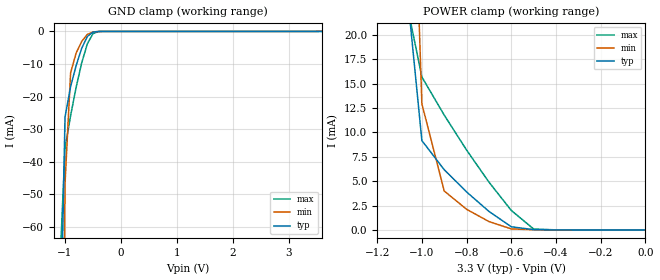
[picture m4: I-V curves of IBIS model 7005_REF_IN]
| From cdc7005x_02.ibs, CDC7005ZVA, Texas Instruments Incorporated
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| Device Control Input Receiver Model REF_IN
[Model]   7005_REF_IN
Model_type  Input
Polarity   Non-Inverting
Vinl = 0.8V
Vinh = 2.0V
| variable   typ   min   max
C_comp   0.57p   NA   NA
[Temperature Range]   27   125   -20
[Voltage range]   3.3   3.0   3.6
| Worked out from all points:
|   GND clamp passes 1 mA (typ) near -0.56 V on its own axis
|   POWER clamp passes 1 mA (typ) near -0.64 V on its own axis
|Process range|   nominal   weak   strong
[POWER Clamp]
|   27C:3.3V:nominal   125C:3.0V:weak   -20C:3.6V:strong
|  Voltage   I(typ)   I(min)   I(max)
-3.6V     4.178A     3.281A     5.394A
-1.1V     32.36mA    81.72mA    26.85mA
-1V       9.154mA    12.92mA    15.67mA
-900mV    6.171mA    3.99mA     11.76mA
-800mV    3.895mA    2.119mA    8.185mA
-700mV    1.902mA    861.1uA    4.902mA
-600mV    327.8uA    109.2uA    1.999mA
-500mV    33.36uA    25.15uA    97.83uA
-400mV    3.107uA    3.538uA    10.35uA
0V        79.56pA    1.099nA    66.3pA
[GND Clamp]
|   27C:3.3V:nominal   125C:3.0V:weak  -20C:3.6V:strong
|  Voltage   I(typ)   I(min)   I(max)
-3.6V     -12.56A    -9.883A    -16.21A
-1.1V     -114.2mA   -281.4mA   -75.16mA
-1V       -26.3mA    -46.85mA   -35.93mA
-900mV    -16.94mA   -12.7mA    -25.87mA
-800mV    -10.42mA   -6.599mA   -17.07mA
-700mV    -5.115mA   -3.041mA   -9.55mA
-600mV    -1.553mA   -923.1uA   -3.791mA
-500mV    -203.4uA   -162.9uA   -687.6uA
-400mV    -13.51uA   -20.23uA   -40.28uA
3.6V      144.4nA    109.2uA    66.3pA
